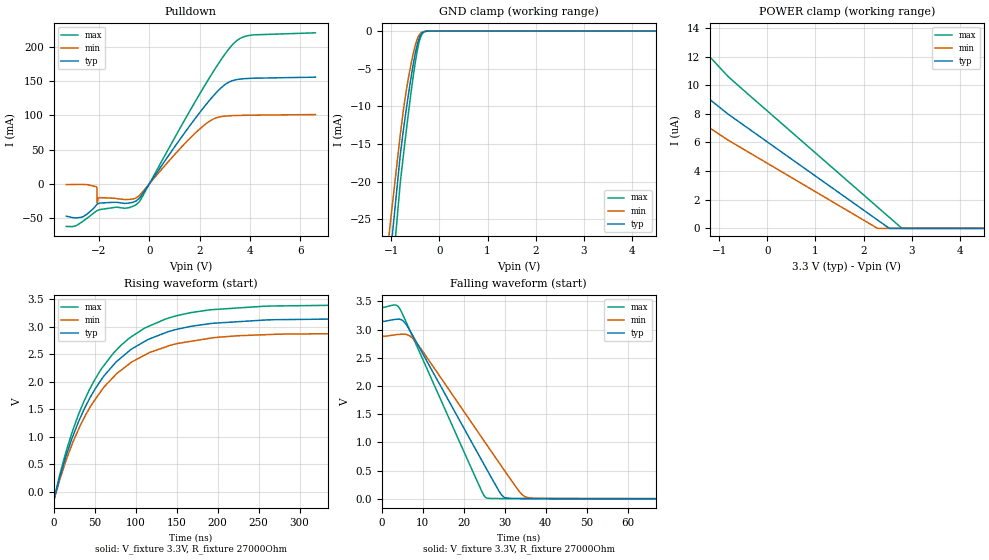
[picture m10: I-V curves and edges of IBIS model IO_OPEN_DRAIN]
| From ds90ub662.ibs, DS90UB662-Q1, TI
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|   IO_OPEN_DRAIN Model
[Model]   IO_OPEN_DRAIN
Model_type   I/O_open_drain
Polarity   Non-Inverting
Enable   Active-Low
Vinl = 0.99
Vinh = 2.31
Vmeas = 1.65
Vref = 3.3
Cref = 1pF
Rref = 27000
|   typ   min   max
C_comp   0.176pF   0.126pF   0.258pF
[Voltage Range]   3.3   3   3.6
[Temperature Range]   27   105   -40
[Pullup Reference]   3.3   3   3.6
[Pulldown Reference]   -0   0   0
[Power Clamp Reference]   3.3   3   3.6
[GND Clamp Reference]   0   0   0
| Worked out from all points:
|   slope of the pulldown table from 0 to 0.495 V, typ, clamps not added: 18.4 ohm
|   GND clamp passes 1 mA (typ) near -0.42 V on its own axis
|   falling waveform, V_fixture 3.3V, R_fixture 27000Ohm: 20-80 % time 14.4ns typ, 16.3ns min, 12.5ns max; typ from 3.15 V to 0.002 V
|   rising waveform, V_fixture 3.3V, R_fixture 27000Ohm: 20-80 % time 74.2ns typ, 75.3ns min, 72.3ns max; typ from 0.002 V to 3.15 V
[Pulldown]
|   Voltage   I(typ)   I(min)   I(max)
-3.3V     -47.2mA    -1.083mA   -62.22mA
-2.676V   -48.56mA   -863.5uA   -55.57mA
-2.102V   -30.79mA   -4.436mA   -39.66mA
-2.082V   -29.95mA   -5.797mA   -39.23mA
-2.072V   -29.62mA   -27.7mA    -39.03mA
-1.983V   -28.19mA   -20.23mA   -37.75mA
-409.2mV  -21.6mA    -17.57mA   -26.53mA
2.095V    108.5mA    83.11mA    137mA
2.927V    142.6mA    98.57mA    185.4mA
3.482V    152.3mA    99.81mA    209.3mA
4.135V    154.2mA    100.3mA    217.5mA
6.6V      155.8mA    101.2mA    220.5mA
[GND Clamp]
|   Voltage   I(typ)   I(min)   I(max)
-3.3V     -395.1mA   -358.4mA   -431.4mA
-1.073V   -34.01mA   -28.65mA   -41.1mA
-1.023V   -29.88mA   -25.55mA   -35.34mA
-815.1mV  -16.47mA   -13.76mA   -20.15mA
-755.7mV  -13.43mA   -10.78mA   -16.84mA
-666.6mV  -9.369mA   -7.031mA   -12.03mA
-557.7mV  -4.897mA   -3.353mA   -6.586mA
-478.5mV  -2.265mA   -1.382mA   -3.226mA
-409.2mV  -767.1uA   -424.1uA   -1.152mA
-349.8mV  -203.3uA   -115.4uA   -303.3uA
-171.6mV  -3.042uA   -2.771uA   -3.369uA
6.6V      0A         0A         0A
[POWER Clamp]
|   Voltage   I(typ)   I(min)   I(max)
-3.3V     21.2uA     14.63uA    63.88uA
-3.142V   19.24uA    13.73uA    51.16uA
-2.449V   14.07uA    10.88uA    23.45uA
-2.34V    13.51uA    10.5uA     21.45uA
-1.845V   11.31uA    8.857uA    15.7uA
-1.498V   9.955uA    7.778uA    13.35uA
-1.34V    9.385uA    7.323uA    12.49uA
-815.1mV  7.974uA    6.16uA     10.6uA
2.284V    602.6nA    14.88nA    1.511uA
2.531V    13.85nA    0A         786nA
2.798V    0A         0A         3.367nA
6.6V      0A         0A         0A
[Ramp]
R_load = 27000
|   typ   min   max
dV/dt_r   1.88543/7.3565e-08   1.7266/7.46981e-08   2.03482/7.21349e-08
dV/dt_f   1.88614/1.43789e-08   1.72733/1.63195e-08   2.0354/1.25056e-08
[Falling Waveform]
V_fixture = 3.3V
V_fixture_min = 3V
V_fixture_max = 3.6V
R_fixture = 27000Ohm
C_fixture = 0F
|   Time   V(typ)   V(min)   V(max)
0s        3.146V     2.881V     3.394V
3.669ns   3.182V     2.91V      3.428V
5.997ns   3.085V     2.912V     3.126V
8.895ns   2.718V     2.726V     2.654V
24.35ns   690.1mV    1.093V     144.6mV
26.24ns   443.5mV    892.6mV    7.46mV
29.87ns   27.89mV    510.9mV    3.486mV
34.22ns   5.385mV    77.27mV    2.766mV
37.38ns   3.442mV    9.621mV    2.634mV
700ns     2.262mV    2.554mV    1.998mV
[Rising Waveform]
V_fixture = 3.3V
V_fixture_min = 3V
V_fixture_max = 3.6V
R_fixture = 27000Ohm
C_fixture = 0F
|   Time   V(typ)   V(min)   V(max)
0s        2.262mV    2.554mV    1.998mV
328.7ps   -17.03mV   659.2uV    -32.39mV
619.8ps   -110.6mV   -121.7mV   -103.4mV
14.42ns   629.9mV    548mV      707.2mV
29.47ns   1.249V     1.114V     1.381V
57ns      2.017V     1.817V     2.21V
91.32ns   2.55V      2.315V     2.781V
136.4ns   2.891V     2.631V     3.138V
256.6ns   3.119V     2.853V     3.369V
700ns     3.145V     2.88V      3.393V
